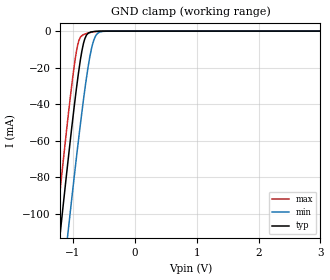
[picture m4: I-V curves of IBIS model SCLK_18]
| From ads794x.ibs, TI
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|   SCLK 1.8V Model
[Model] SCLK_18
Model_type   Input
Vinl = 0.54
Vinh = 1.26
|   typ   min   max
|   (Nom PVT)   (Fast PVT)  (Slow PVT)
C_comp   9.2648480e-13   7.5747950e-13   1.0995770e-12
| POWER = 1.8V
[Model Spec]
Vinl   0.54   0.495   0.6
Vinh   1.26   1.155   1.4
|Vinl = 0.3 X DVDD
|Vinh = 0.7 X DVDD
[Voltage Range]   1.8   1.65   2
[Temperature Range]   27   125   -40
[Power Clamp Reference]   1.8   1.65   2
[GND Clamp Reference]   0   0   0
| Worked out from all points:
|   GND clamp passes 1 mA (typ) near -0.74 V on its own axis
[GND Clamp]
|   Voltage   I(typ)   I(min)   I(max)
-1.8V     -308.6mA   -345.1mA   -287mA
-1.276V   -134.2mA   -173.1mA   -110.5mA
-1.208V   -112.2mA   -151.4mA   -88.18mA
-1.088V   -74.28mA   -113.5mA   -50.27mA
-1.055V   -64.08mA   -103.3mA   -40.24mA
-939.6mV  -30.91mA   -68.63mA   -10.72mA
-901.1mV  -21.17mA   -57.6mA    -5.101mA
-834.8mV  -7.837mA   -39.33mA   -2.022mA
-779.5mV  -2.233mA   -25.65mA   -1.343mA
-691.1mV  -411.9uA   -8.484mA   -566.8uA
-562.9mV  -38.2uA    -510.7uA   -72.75uA
3.595V    0A         0A         0A
[POWER Clamp]
|   SCR cell for ESD function. Effects occurr above VDD x 2
|   Voltage   I(typ)   I(min)   I(max)
-1.8V     0A         0A         0A
0V        0A         0A         0A
3.6V      0A         0A         0A
